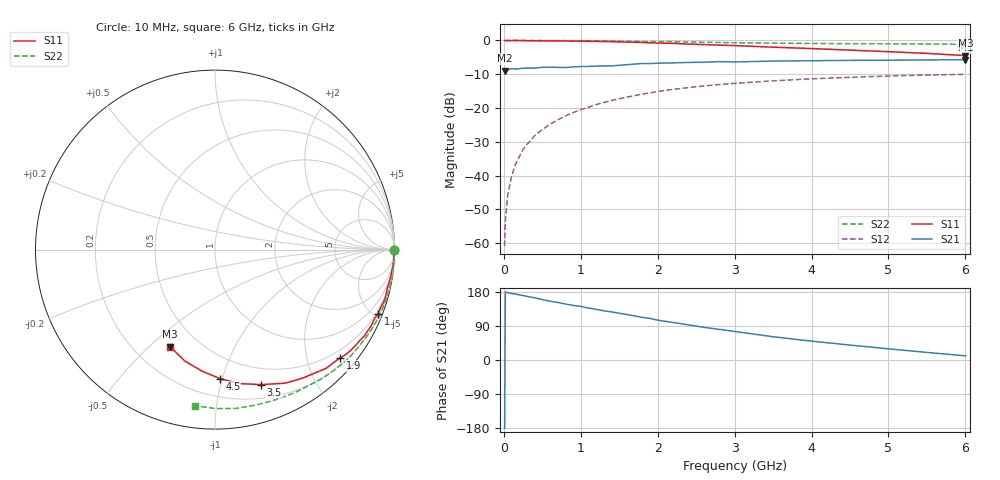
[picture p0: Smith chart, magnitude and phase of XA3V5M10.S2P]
! SIEMENS Discrete & RF Semiconductors
! BFY180
! Si NPN RF Bipolar Junction Transistor in MICRO-X
! VCE = 3.5 V  IC = 0.1 mA
! Common Emitter S-Parameters:  May  1997
# GHz  S  MA  R  50
!  f  S11  S21  S12  S22
! GHz  MAG  ANG  MAG  ANG  MAG  ANG  MAG  ANG
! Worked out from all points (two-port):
!   36 points, 10 MHz to 6 GHz, reference 50 ohm
!   highest |S21| = -5.68 dB at 6 GHz (marker M1); lowest = -8.9 dB at 10 MHz (marker M2)
!   |S21| within 3 dB of the highest: 23.96 MHz to end of sweep
!   lowest |S11| = -4.5 dB at 6 GHz (marker M3), VSWR 3.96, Z = 17.4 - j29.2 ohm
!   |S11| at or under -10 dB: nowhere
!   |S22| runs from -1.1 to 0.0 dB; largest |S21 - S12| = 0.4
!   S11 on the Smith chart (normalised r, x): 10 MHz: open; 1 GHz: 0.34, -5.27; 1.9 GHz: 0.33, -2.65; 3.5 GHz: 0.33, -1.35; 4.5 GHz: 0.33, -0.98; 6 GHz: 0.35, -0.58
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0.01  0.9963 -0.2  0.359 -180.0  0.0009 98.9  0.9984 -0.2
0.02  0.9942 -0.4  0.368 179.2  0.0022 94.7  0.9999 -0.4
0.05  0.994 -0.8  0.369 178.0  0.0051 88.1  0.999 -0.9
0.1  0.9957 -2.1  0.381 175.5  0.0097 90.7  0.9963 -1.9
0.15  0.9994 -3.6  0.379 173.9  0.0146 86.9  0.9999 -2.8
0.25  0.996 -5.5  0.388 170.2  0.0244 85.8  0.9999 -4.7
0.4  0.9905 -8.6  0.39 164.2  0.0389 82.3  0.9989 -7.5
0.5  0.987 -10.9  0.4 159.5  0.0481 80.1  0.9979 -9.4
0.7  0.9858 -15.2  0.399 151.9  0.0668 76.3  0.9955 -13.2
1  0.977 -21.4  0.411 141.5  0.0944 70.1  0.9907 -18.9
1.1  0.9679 -23.5  0.412 137.1  0.1027 68.1  0.9871 -20.7
1.5  0.952 -32.2  0.429 123.3  0.1375 60.1  0.9773 -28.2
1.8  0.9338 -38.8  0.456 112.5  0.1605 54.5  0.9666 -33.7
1.9  0.9228 -40.8  0.454 109.7  0.1675 52.5  0.9641 -35.4
2.2  0.906 -46.9  0.465 98.9  0.189 46.9  0.9567 -40.7
2.8  0.8527 -59.0  0.486 80.8  0.2225 36.4  0.9329 -50.5
3.5  0.7951 -71.1  0.495 61.4  0.2526 25.7  0.9124 -60.9
4  0.7586 -79.8  0.501 49.8  0.2702 18.5  0.9022 -68.1
4.5  0.7191 -87.8  0.507 39.4  0.2845 11.9  0.8957 -75.3
5  0.6819 -95.9  0.51 29.5  0.2975 5.5  0.8926 -82.6
5.5  0.6434 -105.1  0.515 20.0  0.3077 -1.1  0.8856 -89.9
6  0.5965 -114.8  0.52 11.0  0.3145 -7.7  0.8768 -97.2
